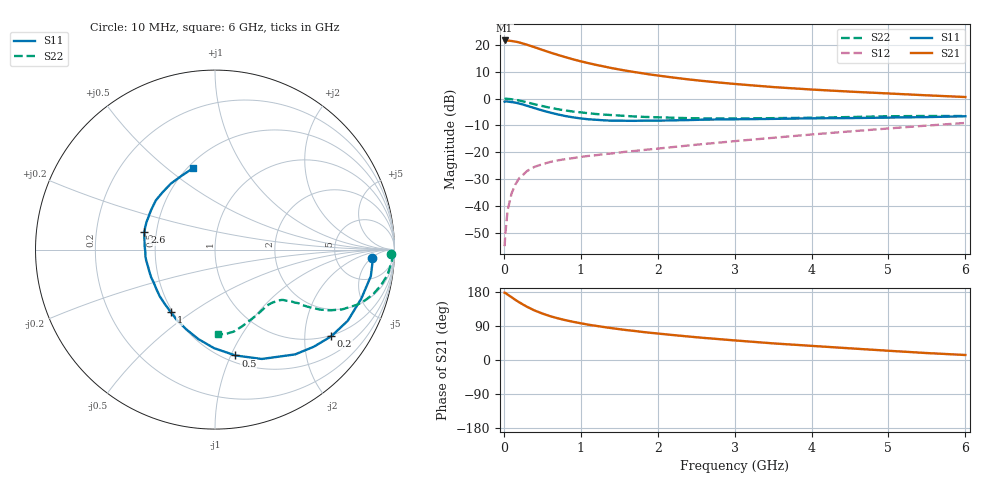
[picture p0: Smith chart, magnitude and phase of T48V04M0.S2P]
! Infineon Technologies  Discrete & RF Semiconductors
! BFR182T
! Si NPN RF Bipolar Junction Transistor in SC75
! VCE = 8 V  IC = 4 mA
! Common Emitter S-Parameters:  October  1999
# GHz  S  MA  R  50
!  f  S11  S21  S12  S22
! GHz  MAG  ANG  MAG  ANG  MAG  ANG  MAG  ANG
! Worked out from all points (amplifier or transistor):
!   36 points, 10 MHz to 6 GHz, reference 50 ohm
!   highest |S21| = 21.6 dB at 10 MHz (marker M1)
!   |S21| within 3 dB of that: start of sweep to 449.3 MHz
!   unconditionally stable (mu >= 1): 1.632 GHz to 4.223 GHz
!   at 250 MHz: K = 0.23, MSG = 24.4 dB, |S12| = -28.4 dB
!   at 1.4 GHz: K = 0.94, MSG = 15.9 dB, |S12| = -20.4 dB
!   at 6 GHz: K = 0.84, MSG = 4.8 dB, |S12| = -9.1 dB
!   S11 on the Smith chart (normalised r, x): 10 MHz: 13, -5; 200 MHz: 0.97, -2.70; 500 MHz: 0.56, -1.04; 1 GHz: 0.49, -0.42; 2.6 GHz: 0.43, +0.10; 6 GHz: 0.53, +0.62
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0.01  0.8734 -2.9  12.02 177.5  0.0018 75.1  0.9836 -1.5
0.02  0.8823 -2.5  11.96 177.1  0.0031 100.3  0.9934 -1.8
0.05  0.8807 -9.7  11.97 172.5  0.0085 90.0  0.9855 -4.3
0.1  0.8597 -18.5  11.74 165.8  0.0171 82.6  0.9712 -8.4
0.15  0.8393 -28.2  11.44 158.7  0.0253 75.7  0.9462 -12.1
0.2  0.808 -36.7  11.05 152.3  0.0331 71.5  0.9177 -15.5
0.3  0.735 -52.6  10.01 140.6  0.0448 64.4  0.8512 -21.1
0.4  0.6629 -66.8  8.999 130.6  0.0537 59.4  0.7827 -25.2
0.5  0.6007 -79.1  8.029 122.7  0.0601 55.8  0.7253 -27.8
0.6  0.5489 -90.6  7.193 115.8  0.066 53.1  0.675 -29.7
0.7  0.5072 -100.5  6.488 110.1  0.0708 52.0  0.6333 -30.9
0.8  0.4725 -109.7  5.885 105.1  0.0747 50.8  0.6008 -31.8
1  0.427 -125.2  4.915 96.9  0.0822 50.4  0.5531 -32.7
1.1  0.4113 -133.4  4.552 93.1  0.0857 50.6  0.5329 -33.6
1.3  0.3934 -146.3  3.95 87.0  0.0925 50.8  0.5032 -34.7
1.6  0.3857 -162.2  3.273 78.8  0.1031 52.6  0.4728 -36.4
2.2  0.3928 176.7  2.458 65.8  0.1254 56.1  0.44 -41.6
2.6  0.4051 166.1  2.115 58.3  0.1429 57.7  0.4277 -45.9
3.5  0.4186 148.3  1.634 43.9  0.1861 59.2  0.4319 -56.8
4.5  0.4328 132.4  1.345 30.8  0.2448 57.9  0.4529 -70.3
5.5  0.4519 114.1  1.147 18.3  0.3141 54.4  0.4737 -82.8
6  0.4689 105.4  1.067 13.2  0.3517 51.4  0.4726 -88.1
